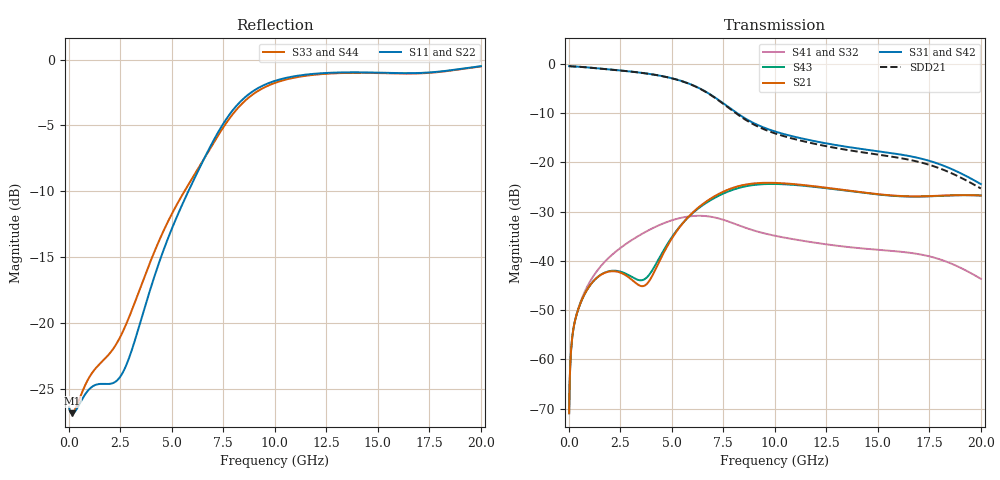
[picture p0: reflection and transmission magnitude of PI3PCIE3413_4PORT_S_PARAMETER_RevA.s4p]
! NPort=4 DATA=800 NOISE=0 GROUPDELAY=0 COMPLEX_DATAFORMAT=POLAR
! NumOfBlock=1 NumOfParam=0
! .MODEL Smodel S TSTONEFILE=PI3PCIE3413_4PORT_S_PARAMETER_RevA.s4p TYPE=S
!  -- The above .MODEL line can be used for the S element in the netlist.
! PORT DEFINITION
! PORT1 = INPUT+
! PORT2 = INPUT-
! PORT3 = OUTPUT+
! PORT4 = OUTPUT-
# Hz S MA R  50
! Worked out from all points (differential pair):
!   800 points, 25 MHz to 20 GHz, reference 50 ohm
!   strongest paths, dB at 25 MHz, 5.025 GHz, 10.03 GHz, 15.03 GHz, 20 GHz:
!     S31: -0.5, -2.9, -13.7, -17.7, -24.4
!     S42: -0.5, -2.9, -13.7, -17.7, -24.4
!     S21: -70.9, -35.3, -24.2, -26.5, -26.7
!     S43: -70.9, -35.1, -24.4, -26.5, -26.7
!     S41: -70.9, -31.7, -34.9, -37.7, -43.6
!     S32: -70.9, -31.7, -34.9, -37.7, -43.6
!   taken as a pair (ports 1,2 in; 3,4 out), SDD21 dB: -0.5, -3.0, -14.1, -18.4, -25.3
!   lowest |S11| = -26.9 dB at 175 MHz (marker M1), VSWR 1.10, Z = 54.8 - j0.00384 ohm
!   |S11| at or under -10 dB: start of sweep to 5.811 GHz
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2.5e7  0.04782 -2.4  0.0002849 85.9  0.9468 -0.8  0.0002842 85.9
       0.0002849 85.9  0.04782 -2.4  0.0002842 85.9  0.9469 -0.8
       0.9469 -0.8  0.0002842 85.9  0.04784 -2.0  0.0002849 86.0
       0.0002842 85.9  0.9469 -0.8  0.0002849 86.0  0.04784 -2.0
1.75e8  0.04536 -0.0  0.001671 69.1  0.9428 -4.4  0.001671 68.9
        0.001671 69.1  0.04536 -0.1  0.001671 68.9  0.9428 -4.4
        0.9428 -4.4  0.001671 68.9  0.04563 2.5  0.001671 69.2
        0.001671 68.9  0.9428 -4.4  0.001671 69.2  0.04563 2.5
1.325e9  0.05822 -6.3  0.006611 53.4  0.9038 -31.3  0.007646 50.0
         0.006612 53.4  0.05813 -6.4  0.007646 50.0  0.9038 -31.3
         0.9039 -31.3  0.007646 50.0  0.0674 4.6  0.006622 54.5
         0.007647 50.0  0.9038 -31.3  0.006622 54.5  0.06731 4.5
3.25e9  0.08756 8.0  0.005983 51.5  0.8246 -74.3  0.01722 12.9
        0.005983 51.5  0.08732 8.1  0.01722 12.9  0.8245 -74.4
        0.8247 -74.3  0.01722 13.0  0.1217 5.2  0.006566 55.1
        0.01722 13.0  0.8246 -74.3  0.006566 55.1  0.1215 5.2
6.125e9  0.3562 -13.5  0.03244 93.3  0.5944 -144.8  0.02864 -60.4
         0.03244 93.3  0.3561 -13.5  0.02864 -60.4  0.5942 -144.8
         0.5945 -144.8  0.02865 -60.4  0.3677 -21.9  0.03194 88.9
         0.02865 -60.4  0.5943 -144.8  0.03194 88.9  0.3675 -21.8
1.0825e10  0.8604 -82.3  0.06045 15.2  0.1848 155.4  0.01671 -151.7
           0.06045 15.2  0.8606 -82.3  0.01671 -151.7  0.1847 155.4
           0.1849 155.5  0.01672 -151.6  0.8493 -82.8  0.05931 15.4
           0.01672 -151.6  0.1847 155.5  0.05931 15.4  0.8495 -82.8
2e10  0.9435 -125.0  0.04617 -28.2  0.06018 27.2  0.006578 52.0
      0.04617 -28.2  0.9435 -125.0  0.006578 52.0  0.06018 27.2
      0.06024 27.3  0.006584 52.1  0.9413 -125.0  0.04608 -27.9
      0.006584 52.1  0.06023 27.3  0.04608 -27.9  0.9413 -125.0
